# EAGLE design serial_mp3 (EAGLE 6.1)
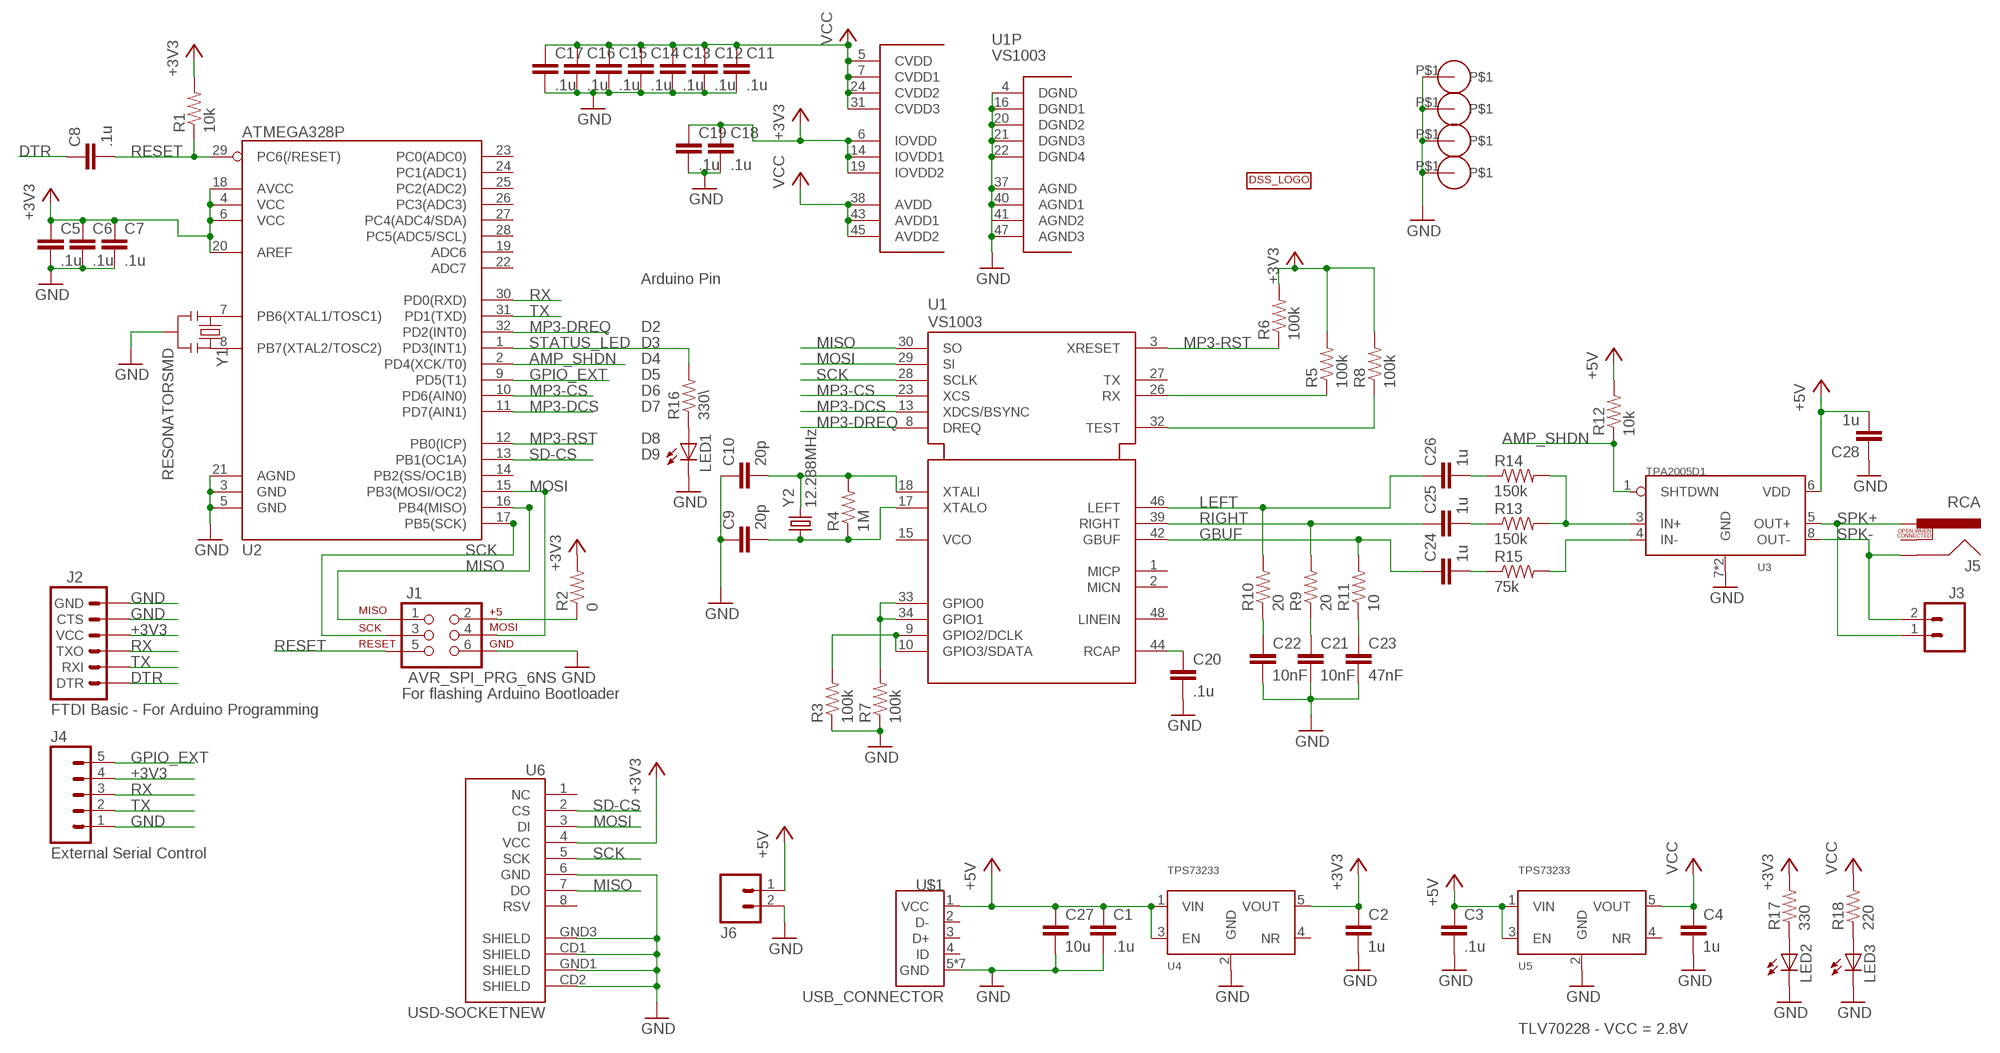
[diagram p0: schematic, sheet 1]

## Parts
C1  .1u  CAP0603-CAP  [0603-CAP]
C2  1u  CAP0603-CAP  [0603-CAP]
C3  .1u  CAP0603-CAP  [0603-CAP]
C4  1u  CAP0603-CAP  [0603-CAP]
C5  .1u  CAP0603-CAP  [0603-CAP]
C6  .1u  CAP0603-CAP  [0603-CAP]
C7  .1u  CAP0603-CAP  [0603-CAP]
C8  .1u  CAP0603-CAP  [0603-CAP]
C9  20p  CAP0603-CAP  [0603-CAP]
C10  20p  CAP0603-CAP  [0603-CAP]
C11  .1u  CAP0603-CAP  [0603-CAP]
C12  .1u  CAP0603-CAP  [0603-CAP]
C13  .1u  CAP0603-CAP  [0603-CAP]
C14  .1u  CAP0603-CAP  [0603-CAP]
C15  .1u  CAP0603-CAP  [0603-CAP]
C16  .1u  CAP0603-CAP  [0603-CAP]
C17  .1u  CAP0603-CAP  [0603-CAP]
C18  .1u  CAP0603-CAP  [0603-CAP]
C19  .1u  CAP0603-CAP  [0603-CAP]
C20  .1u  CAP0603-CAP  [0603-CAP]
C21  10nF  CAP0603-CAP  [0603-CAP]
C22  10nF  CAP0603-CAP  [0603-CAP]
C23  47nF  CAP0603-CAP  [0603-CAP]
C24  1u  CAP0603-CAP  [0603-CAP]
C25  1u  CAP0603-CAP  [0603-CAP]
C26  1u  CAP0603-CAP  [0603-CAP]
C27  10u  CAP0603-CAP  [0603-CAP]
C28  1u  CAP0603-CAP  [0603-CAP]
J1  AVR_SPI_PRG_6NS  [2X3-NS]
J2  ARDUINO_SERIAL_PROGRAMPTH  [1X06]
J3  M02PTH  [1X02]
J4  M05PTH  [1X05]
J5  RCA  [RCA]
J6  M02PTH  [1X02]
LED1  LED0603  [LED-0603]
LED2  LED0603  [LED-0603]
LED3  LED0603  [LED-0603]
R1  10k  RESISTOR0603-RES  [0603-RES]
R2  0  RESISTOR0603-RES  [0603-RES]
R3  100k  RESISTOR0603-RES  [0603-RES]
R4  1M  RESISTOR0603-RES  [0603-RES]
R5  100k  RESISTOR0603-RES  [0603-RES]
R6  100k  RESISTOR0603-RES  [0603-RES]
R7  100k  RESISTOR0603-RES  [0603-RES]
R8  100k  RESISTOR0603-RES  [0603-RES]
R9  20  RESISTOR0603-RES  [0603-RES]
R10  20  RESISTOR0603-RES  [0603-RES]
R11  10  RESISTOR0603-RES  [0603-RES]
R12  10k  RESISTOR0603-RES  [0603-RES]
R13  150k  RESISTOR0603-RES  [0603-RES]
R14  150k  RESISTOR0603-RES  [0603-RES]
R15  75k  RESISTOR0603-RES  [0603-RES]
R16  330\  RESISTOR0603-RES  [0603-RES]
R17  330  RESISTOR0603-RES  [0603-RES]
R18  220  RESISTOR0603-RES  [0603-RES]
U1  VS1003  [LQFP48]
U2  ATMEGA328P  ATMEGA328_SMT  [TQFP32-08]
U3  TPA2005D1  [S-PDSO-G08]
U4  TPS73233  [SOT23-5]
U5  TPS73233  [SOT23-5]
U6  USD-SOCKETNEW  [MICRO-SD-SOCKET-PP]
U$1  USB_CONNECTOR  [USB_MICRO]
U$2  DSSTOP  [DSS]
U$3  GNDHOLE  [GNDHOLE]
U$4  GNDHOLE  [GNDHOLE]
U$5  GNDHOLE  [GNDHOLE]
U$6  GNDHOLE  [GNDHOLE]
Y1  RESONATORSMD  [RESONATOR-SMD]
Y2  12.288MHz  NX3225GA  [SMD-4_3]

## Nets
+3V3: C2.1 C5.1 C6.1 C7.1 C18.1 C19.1 J2.4(VCC) J4.4 R1.2 R2.2 R5.2 R6.2 R8.2 R17.2 U1.6(IOVDD) U1.14(IOVDD1) U1.19(IOVDD2) U2.4(VCC) U2.6(VCC) U2.18(AVCC) U2.20(AREF) U4.5(VOUT) U6.4(VCC)
+5V: C1.1 C3.1 C27.1 C28.2 J6.1 R12.2 U3.6(VDD) U4.1(VIN) U4.3(EN) U5.1(VIN) U5.3(EN) U$1.1(VCC)
AMP_SHDN: R12.1 U2.2(PD4(XCK/T0)) U3.1(SHTDWN)
DTR: C8.1 J2.1(DTR)
GBUF: C24.1 R11.2 U1.42(GBUF)
GND: C1.2 C2.2 C3.2 C4.2 C5.2 C6.2 C7.2 C9.1 C10.1 C11.2 C12.2 C13.2 C14.2 C15.2 C16.2 C17.2 C18.2 C19.2 C20.2 C21.2 C22.2 C23.2 C27.2 C28.1 J1.6 J2.5(CTS) J2.6(GND) J4.1 J6.2 LED1.C LED2.C LED3.C R3.1 R7.1 U1.4(DGND) U1.16(DGND1) U1.20(DGND2) U1.21(DGND3) U1.22(DGND4) U1.37(AGND) U1.40(AGND1) U1.41(AGND2) U1.47(AGND3) U2.3(GND) U2.5(GND) U2.21(AGND) U3.7(GND) U3.TH(GND) U4.2(GND) U5.2(GND) U6.6(GND) U6.CD1(SHIELD) U6.CD2(SHIELD) U6.GND1(SHIELD) U6.GND3(SHIELD) U$1.5(GND) U$1.GND1(GND) U$1.GND2(GND) U$1.GND3(GND) U$1.GND4(GND) U$1.GND5(GND) U$1.GND6(GND) U$3.P$1 U$4.P$1 U$5.P$1 U$6.P$1 Y1.2
GPIO_EXT: J4.5 U2.9(PD5(T1))
LEFT: C26.1 R10.2 U1.46(LEFT)
MISO: J1.1 U1.30(SO) U2.16(PB4(MISO)) U6.7(DO)
MOSI: J1.4 U1.29(SI) U2.15(PB3(MOSI/OC2)) U6.3(DI)
MP3-CS: U1.23(XCS) U2.10(PD6(AIN0))
MP3-DCS: U1.13(XDCS/BSYNC) U2.11(PD7(AIN1))
MP3-DREQ: U1.8(DREQ) U2.32(PD2(INT0))
MP3-RST: R6.1 U1.3(XRESET) U2.12(PB0(ICP))
N$1: J1.2 R2.1
N$2: C10.2 R4.2 U1.18(XTALI) Y2.3
N$3: C9.2 R4.1 U1.17(XTALO) Y2.1
N$4: R7.2 U1.33(GPIO0) U1.34(GPIO1)
N$5: U2.8(PB7(XTAL2/TOSC2)) Y1.3
N$6: U2.7(PB6(XTAL1/TOSC1)) Y1.1
N$7: R5.1 U1.26(RX)
N$8: R8.1 U1.32(TEST)
N$9: C20.1 U1.44(RCAP)
N$10: C23.1 R11.1
N$11: C22.1 R10.1
N$12: C21.1 R9.1
N$13: C24.2 R15.1
N$14: C25.2 R13.1
N$15: C26.2 R14.1
N$16: R13.2 R14.2 U3.3(IN+)
N$17: R15.2 U3.4(IN-)
N$18: R3.2 U1.9(GPIO2/DCLK) U1.10(GPIO3/SDATA)
N$20: LED2.A R17.1
N$21: LED1.A R16.1
N$22: LED3.A R18.1
RESET: C8.2 J1.5 R1.1 U2.29(PC6(/RESET))
RIGHT: C25.1 R9.2 U1.39(RIGHT)
RX: J2.3(TXO) J4.3 U2.30(PD0(RXD))
SCK: J1.3 U1.28(SCLK) U2.17(PB5(SCK)) U6.5(SCK)
SD-CS: U2.13(PB1(OC1A)) U6.2(CS)
SPK+: J3.1 J5.PIN U3.5(OUT+)
SPK-: J3.2 J5.SHELL U3.8(OUT-)
STATUS_LED: R16.2 U2.1(PD3(INT1))
TX: J2.2(RXI) J4.2 U2.31(PD1(TXD))
VCC: C4.1 C11.1 C12.1 C13.1 C14.1 C15.1 C16.1 C17.1 R18.2 U1.5(CVDD) U1.7(CVDD1) U1.24(CVDD2) U1.31(CVDD3) U1.38(AVDD) U1.43(AVDD1) U1.45(AVDD2) U5.5(VOUT)
Unconnected: J5.SWITCH U1.1(MICP) U1.2(MICN) U1.15(VCO) U1.27(TX) U1.48(LINEIN) U2.14(PB2(SS/OC1B)) U2.19(ADC6) U2.22(ADC7) U2.23(PC0(ADC0)) U2.24(PC1(ADC1)) U2.25(PC2(ADC2)) U2.26(PC3(ADC3)) U2.27(PC4(ADC4/SDA)) U2.28(PC5(ADC5/SCL)) U4.4(NR) U5.4(NR) U6.1(NC) U6.8(RSV) U$1.2(D-) U$1.3(D+) U$1.4(ID)

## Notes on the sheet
- Arduino Pin
- D2
- D3
- D4
- D5
- D6
- D7
- D8
- D9
- For flashing Arduino Bootloader
- FTDI Basic - For Arduino Programming
- External Serial Control
- TLV70228 - VCC = 2.8V

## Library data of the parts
C1-C28 = SparkFun-Passives:CAP: Capacitor
J1 = SparkFun-Connectors:AVR_SPI_PRG_6: AVR ISP 6 Pin This is the reduced ISP connector for AVR programming. Common on Arduino. This footprint will take up less PCB space and can be used with a 10-pin to 6-pin adapter such as SKU: BOB-08508
J2 = SparkFun-Connectors:ARDUINO_SERIAL_PROGRAM: FTDI connector footprints
J3 J6 = SparkFun-Connectors:M02: Header 2
J4 = SparkFun-Connectors:M05: Header 5 Standard 5-pin 0.1" header. Use with straight break away headers (SKU : PRT-00116), right angle break away headers (PRT-00553), swiss pins (PRT-00743), machine pins (PRT-00117), and female headers (PRT-00115). Molex polarized connector foot print use with SKU : PRT-08230 with associated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
J5 = SparkFun-Connectors:RCA
LED1-LED3 = SparkFun-LED:LED: LEDs
R1-R18 = SparkFun-Passives:RESISTOR: Resistor
U1 = vlsi-web:VS1003: MP3 / WMA / MIDI Audio Codec Circuit
U2 = SparkFun-DigitalIC:ATMEGA328_SMT: 32-Pin Atmega328 part Commonly used on Arduino compatible boards Available in QFP and QFN packages TQFP is IC-09069 QFN is non-stock; PROD_ID: IC-09069
U3 = DSS:TPA2005D1: TI TPA2005D1 1.4 W mono class D audio amp
U4 U5 = DSS:TPS73233: TI TPS73233 - fixed output http://www.ti.com/product/tps73233
U6 = SparkFun-Connectors:USD-SOCKET: microSD Socket Push-push type uSD socket. Schematic element and footprint production proven. Spark Fun Electronics SKU : PRT-00127. tDoc lines correctly indicate media card edge positions when inserting (unlocked, locked, depressed).
U$1 = DSS:USB_CONNECTOR: USB Connector http://www.digikey.com/product-detail/en/10118192-0001LF/609-4613-1-ND/2785378
U$2 = DSS:DSS: DSS LOGO
U$3-U$6 = GT-IEEE:GNDHOLE
Y1 = SparkFun-FreqCtrl:RESONATOR: Resonator Small SMD resonator. This is the itty bitty 10/20MHz resonators with built in caps. CSTCE10M0G55 and CSTCE20M0V53. Footprint has been reviewed closely but hasn't been tested yet.
Y2 = DSS:NX3225GA: NX3225GA 26 MHz SMD crystal

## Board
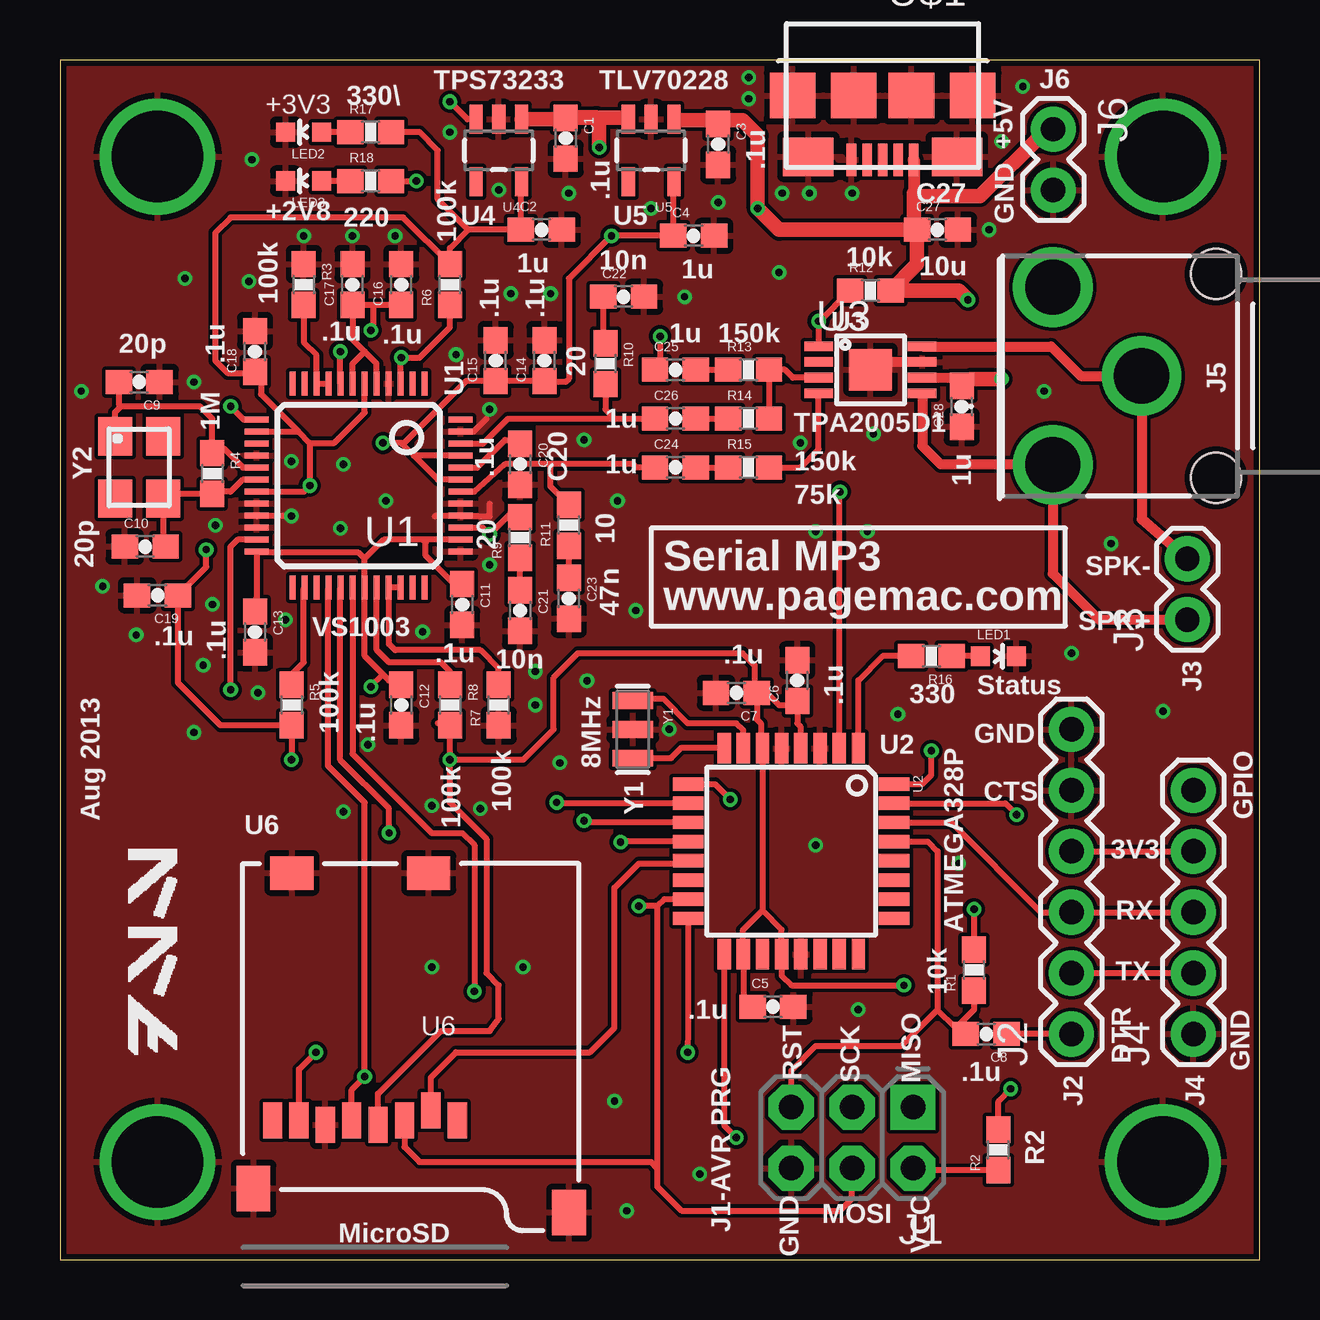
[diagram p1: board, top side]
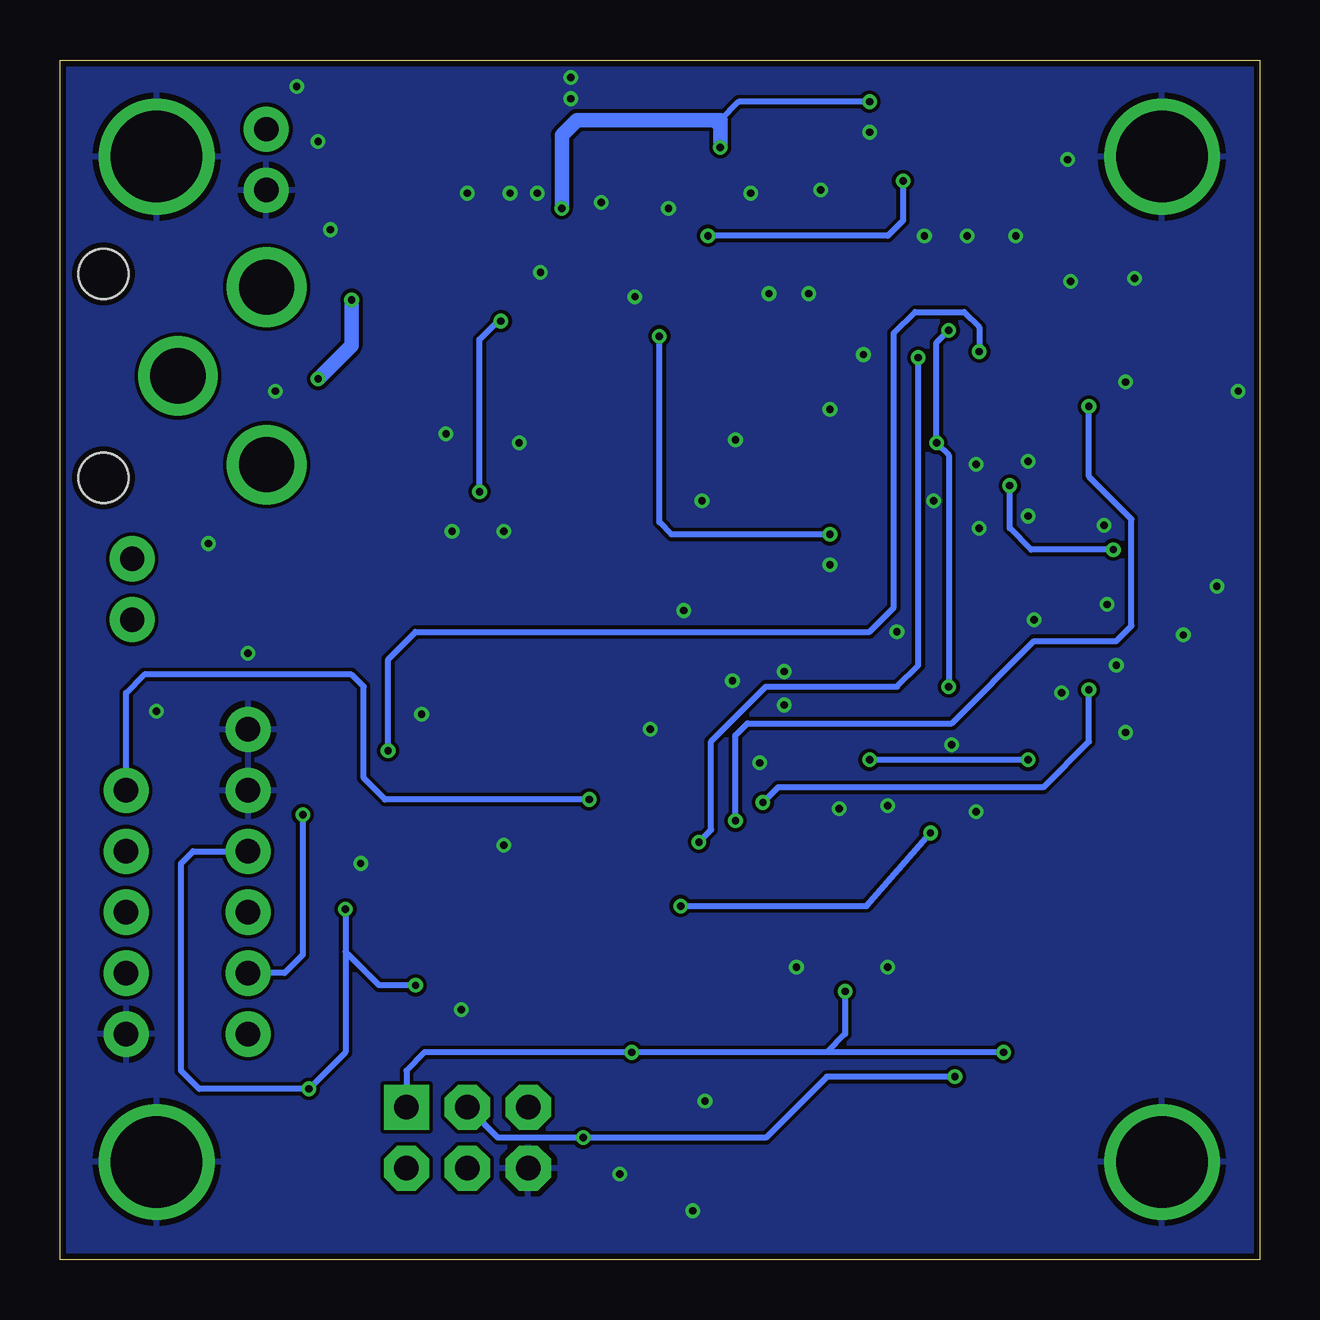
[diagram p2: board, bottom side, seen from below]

Size 50 x 50 mm. Coordinates in mm from the lower left corner, seen from the top.
Outline: 0,0 50,0 50,50 0,50 0,0
Copper layers (1*16): Top 0.035mm / dielectric 1.5mm / Bottom 0.035mm
Design rules: minimum track width 6mil, minimum drill 12mil, track to track 6mil, track to pad 6mil, pad to pad 6mil, via to via 6mil, smd to smd 0mil, copper to edge 10mil, drill to drill 10mil, minimum pad ring 10mil, minimum via ring 6mil, stop-mask expansion 2mil, vias tented up to drill 100mil, thermal gap 10mil

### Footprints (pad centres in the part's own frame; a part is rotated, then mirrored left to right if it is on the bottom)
0603-CAP = smd 1.1 x 1: 1 -0.85,0; 2 0.85,0
2X3-NS = drill 1.016 pad 1.88 square: 1 -2.54,-1.27 | drill 1.016 pad 1.88 octagon: 2 -2.54,1.27; 3 0,-1.27; 4 0,1.27; 5 2.54,-1.27; 6 2.54,1.27
1X06 = drill 1.016 pad 1.88: 1 0,0; 2 2.54,0; 3 5.08,0; 4 7.62,0; 5 10.16,0; 6 12.7,0
1X02 = drill 1.016 pad 1.88: 1 0,0; 2 2.54,0
1X05 = drill 1.016 pad 1.88: 1 0,0; 2 2.54,0; 3 5.08,0; 4 7.62,0; 5 10.16,0
RCA = drill 2.3: PIN 3.7,3.7; SHELL 0,0; SWITCH 3.7,-3.7 | hole 2.1: -3.1,4.25; -3.1,-4.25
LED-0603 = smd 0.8 x 0.8: A 0,-0.75; C 0,0.75
0603-RES = smd 1.1 x 1: 1 -0.85,0; 2 0.85,0
LQFP48 = smd 0.25 x 1: 1 -2.75,-4.25; 2 -2.25,-4.25; 3 -1.75,-4.25; 4 -1.25,-4.25; 5 -0.75,-4.25; 6 -0.25,-4.25; 7 0.25,-4.25; 8 0.75,-4.25; 9 1.25,-4.25; 10 1.75,-4.25; 11 2.25,-4.25; 12 2.75,-4.25; 25 2.75,4.25; 26 2.25,4.25; 27 1.75,4.25; 28 1.25,4.25; 29 0.75,4.25; 30 0.25,4.25; 31 -0.25,4.25; 32 -0.75,4.25; 33 -1.25,4.25; 34 -1.75,4.25; 35 -2.25,4.25; 36 -2.75,4.25 | smd 1 x 0.25: 13 4.25,-2.75; 14 4.25,-2.25; 15 4.25,-1.75; 16 4.25,-1.25; 17 4.25,-0.75; 18 4.25,-0.25; 19 4.25,0.25; 20 4.25,0.75; 21 4.25,1.25; 22 4.25,1.75; 23 4.25,2.25; 24 4.25,2.75; 37 -4.25,2.75; 38 -4.25,2.25; 39 -4.25,1.75; 40 -4.25,1.25; 41 -4.25,0.75; 42 -4.25,0.25; 43 -4.25,-0.25; 44 -4.25,-0.75; 45 -4.25,-1.25; 46 -4.25,-1.75; 47 -4.25,-2.25; 48 -4.25,-2.75
TQFP32-08 = smd 1.27 x 0.559: 1 -4.293,2.8; 2 -4.293,2; 3 -4.293,1.2; 4 -4.293,0.4; 5 -4.293,-0.4; 6 -4.293,-1.2; 7 -4.293,-2; 8 -4.293,-2.8; 17 4.293,-2.8; 18 4.293,-2; 19 4.293,-1.2; 20 4.293,-0.4; 21 4.293,0.4; 22 4.293,1.2; 23 4.293,2; 24 4.293,2.8 | smd 0.559 x 1.27: 9 -2.8,-4.293; 10 -2,-4.293; 11 -1.2,-4.293; 12 -0.4,-4.293; 13 0.4,-4.293; 14 1.2,-4.293; 15 2,-4.293; 16 2.8,-4.293; 25 2.8,4.293; 26 2,4.293; 27 1.2,4.293; 28 0.4,4.293; 29 -0.4,4.293; 30 -1.2,4.293; 31 -2,4.293; 32 -2.8,4.293
S-PDSO-G08 = smd 0.4 x 1.2: 1 -0.975,-2.157; 2 -0.325,-2.157; 3 0.325,-2.157; 4 0.975,-2.157; 5 0.975,2.157; 6 0.325,2.157; 7 -0.325,2.157; 8 -0.975,2.157 | smd 1.73 x 1.78: TH 0,0
SOT23-5 = smd 0.55 x 1.2: 1 -0.95,-1.3; 2 0,-1.3; 3 0.95,-1.3; 4 0.95,1.3; 5 -0.95,1.3
MICRO-SD-SOCKET-PP = smd 0.8 x 1.5: 1 -8.94,10.7; 2 -7.84,10.3; 3 -6.74,10.7; 4 -5.64,10.9; 5 -4.54,10.7; 6 -3.44,10.9; 7 -2.34,10.7; 8 -1.24,10.7 | smd 1.8 x 1.4: CD1 -2.05,0.4; CD2 -7.75,0.4 | smd 1.4 x 1.9: GND1 -13.6,14.55; GND3 -0.45,13.55
USB_MICRO = smd 0.4 x 1.35: 1 -1.3,2.675; 2 -0.65,2.675; 3 0,2.675; 4 0.65,2.675; 5 1.3,2.675 | smd 1.9 x 1.9: GND1 -3.75,0; GND2 -1.2,0; GND3 1.2,0; GND4 3.75,0 | smd 2.1 x 1.6: GND5 -3.1,2.55; GND6 3.1,2.55
GNDHOLE = drill 3.81: P$1 0,0
RESONATOR-SMD = smd 0.7 x 1.7: 1 -1.2,0; 2 0,0; 3 1.2,0
SMD-4_3 = smd 1.6 x 1.4: 1 -1.3,-1; 2 1.3,-1; 3 1.3,1; 4 -1.3,1

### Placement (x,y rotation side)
C1  21.08,46.74 270 top
C2  20.07,42.93 0 top
C3  27.43,46.48 270 top
C4  26.42,42.67 0 top
C5  29.72,10.54 0 top
C6  30.73,24.13 90 top
C7  28.19,23.62 180 top
C8  38.61,9.4 180 top
C9  3.3,36.58 180 top
C10  3.56,29.72 0 top
C11  16.76,27.3 270 top
C12  14.22,23.11 270 top
C13  8.13,26.16 270 top
C14  20.19,37.47 90 top
C15  18.16,37.47 90 top
C16  14.22,40.64 90 top
C17  12.19,40.64 90 top
C18  8.13,37.85 90 top
C19  4.06,27.69 180 top
C20  19.18,33.15 270 top
C21  19.18,27.05 270 top
C22  23.5,40.13 0 top
C23  21.21,27.56 270 top
C24  25.65,33.02 0 top
C25  25.65,37.08 0 top
C26  25.65,35.05 0 top
C27  36.58,42.93 0 top
C28  37.59,35.56 90 top
J1  33.02,5.08 180 top
J2  42.16,9.4 90 top
J3  46.99,26.67 90 top
J4  47.24,9.4 90 top
J5  45.09,36.83 180 top
J6  41.4,47.12 270 top
LED1  39.12,25.15 270 top
LED2  10.16,46.99 90 top
LED3  10.16,44.96 90 top
R1  38.1,12.06 90 top
R2  39.12,4.57 90 top
R3  10.16,40.64 270 top
R4  6.35,32.77 270 top
R5  9.65,23.11 270 top
R6  16.26,40.64 90 top
R7  18.29,23.11 90 top
R8  16.26,23.11 270 top
R9  19.18,30.1 90 top
R10  22.73,37.34 270 top
R11  21.21,30.61 90 top
R12  33.78,40.39 0 top
R13  28.7,37.08 0 top
R14  28.7,35.05 0 top
R15  28.7,33.02 0 top
R16  36.32,25.15 180 top
R17  12.95,46.99 0 top
R18  12.95,44.96 0 top
U1  12.45,32.26 180 top
U2  30.48,17.02 270 top
U3  33.78,37.08 270 top
U4  18.29,46.23 180 top
U5  24.64,46.23 180 top
U6  7.62,16.51 180 top
U$1  34.29,48.51 180 top
U$2  5.08,8.38 90 top
U$3  45.97,4.06 0 top
U$4  4.06,4.06 0 top
U$5  4.06,45.97 0 top
U$6  45.97,45.97 0 top
Y1  23.88,22.1 270 top
Y2  3.3,33.02 270 top

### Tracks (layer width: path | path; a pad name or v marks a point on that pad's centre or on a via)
+3V3  (via drill 0.3)
  Top 0.254: 29.28,14.55 U2.6 29.21,21.38 29.21,22.35 29.04,22.52 C7.1 29.08,23.62 | 29.28,14.55 28.45,13.72 28.45,12.76 U2.18 28.48,10.68 C5.1 | 29.28,14.55 30.08,13.75 U2.20 30.08,11.83 30.48,11.43 v35.18,11.43 | J2.4 J4.4 | R2.2 39.12,6.6 v39.62,7.11 | v38.1,14.61 R1.2 38.1,12.83 | U1.14 9.94,34.51 | 9.94,34.51 10.41,34.04 | 10.41,34.04 v10.41,32.26 10.16,32 U1.19 | 10.41,34.04 11.43,34.04 12.7,35.31 U1.6 | U6.4 13.26,6.91 15.88,9.53 17.91,9.53 18.29,10.03 18.29,11.43 17.78,11.94 17.78,17.53 16.26,19.05 v16.26,20.83 | U4.5 19.22,44.91 C2.1 17.02,42.93 | 17.02,42.93 15.75,44.2 15.75,46.23 14.99,46.99 R17.2 | v9.65,20.83 R5.2 6.69,22.26 4.91,24.04 C19.1 6.1,28.87 v6.1,29.59 | 15.75,22.35 R8.2 v16.26,20.83 | 17.02,42.93 16.26,42.16 R6.2 14.31,43.43 7.11,43.43 6.48,42.8 6.48,37.47 6.99,36.96 8.38,36.96 | U2.4 30.86,21.33 30.86,22.23 30.73,22.35 C6.1 30.57,23.11 29.97,23.11 29.46,23.62 29.08,23.62 | C18.1 8.38,36.96 | 8.38,36.96 8.38,36.07 9.94,34.51 | v16.26,20.83 19.3,20.83 20.57,22.1 20.57,24.26 21.59,25.27 28.45,25.27 28.96,24.77 28.96,23.75 29.08,23.62
  Bottom 0.254: J2.4 44.45,17.02 44.96,16.51 44.96,7.87 44.2,7.11 v39.62,7.11 38.1,8.64 38.1,12.83 | v38.1,14.61 38.1,12.83 | v6.1,29.59 9.53,29.59 10.41,30.48 v10.41,32.26 | v9.65,20.83 v16.26,20.83 | v35.18,11.43 36.7,11.43 38.1,12.83
+5V  (via drill 0.3)
  Top 0.254: 35.59,43.32 C27.1 | 27.6,47.5 C3.1 | 21.08,47.5 21.05,47.53 21.05,47.56 C1.1 | 23.63,47.59 U5.3 | J6.1 41.02,46.99 | 35.72,44.32 35.59,44.45 | U4.3 16.99,47.53 v16.26,48.26 | 25.65,47.5 25.62,47.5 U5.1
  Top 0.406: U3.6 38.01,36.76 C28.2
  Top 0.508: U$1.1 35.59,44.45
  Top 0.61: 35.59,44.45 35.59,43.32 | 27.6,47.5 28.45,47.5 29.08,46.86 v29.08,43.81 29.97,42.93 C27.1 35.73,41.48 R12.2 37.47,40.39 v37.85,40.01 | U4.1 21.05,47.53 | 23.63,47.59 C1.1 21.12,47.62 22.35,47.62 22.48,47.5 v22.48,46.35 | 41.02,46.99 38.35,44.32 35.72,44.32 | C3.1 27.27,47.5 25.65,47.5 | v39.24,36.7 37.97,36.7 C28.2
  Bottom 0.254: v16.26,48.26 21.72,48.26 22.48,47.5 22.73,47.24
  Bottom 0.61: v22.48,46.35 22.48,47.5 28.45,47.5 29.08,46.86 v29.08,43.81 | v37.85,40.01 37.85,38.1 v39.24,36.7
AMP_SHDN  (via drill 0.3)
  Top 0.254: U3.1 31.62,39.08 | 31.62,39.08 R12.1 | U2.2 32.48,31.97 v32.51,32 | 31.62,39.08 v31.62,39.11 v31.62,39.12
  Bottom 0.254: v32.51,32 32.51,38.35 31.71,39.16 31.67,39.16 v31.62,39.12
DTR
  Top 0.254: J2.1 C8.1
GBUF
  Top 0.254: U1.42 17.28,32.01 18.54,33.15 20.45,33.15 | C24.1 24,33.02 23.88,33.15 20.45,33.15 | R11.2 20.45,32.22 20.45,33.15
GND  (via drill 0.3)
  Top 0.254: U1.47 17.24,34.51 17.78,35.05 | v9.65,30.99 8.22,30.99 U1.21 | U1.40 16.72,30.99 | 16.72,30.99 17.91,30.99 17.91,31.5 | 16.72,30.99 15.62,30.99
  Top 0.406: U3.7 33.98,37.41 U3.TH
  other vias: 19.3,12.19 7.87,40.77 33.66,30.35 23.11,6.6 33.27,10.41 37.47,16.51 8,45.85 5.21,40.89 38.73,42.93 29.97,41.15 20.83,20.7 31.5,17.27 45.97,22.86 3.17,26.04 23.62,2.03 15.49,18.92 25.4,22.1 15.49,12.19 9.65,33.27 13.59,31.62 15.11,26.16 21.97,24.13 30.86,34.04 21.84,34.16 23.24,31.62 17.91,35.43 20.45,40.26 18.8,40.26 13.97,42.67 12.19,42.67 10.16,42.67 31.24,44.45 28.7,49.28 39.24,46.61 6.48,30.61 6.35,27.3 1.78,28.07 5.59,36.58 0.89,36.2 8.26,23.62 21.21,44.45 18.29,44.58 16.26,46.99 24.64,43.81 27.43,44.07 26.04,40.13 12.83,21.46 17.53,18.8 26.67,3.56 19.81,24.51 24,27.05 17.91,28.96 11.81,33.15 16.51,37.72 5.59,21.97 11.81,18.67 11.68,30.48 5.97,24.77 41.02,36.2 31.5,30.35 43.81,29.84 42.16,25.27 34.92,22.73 33.02,44.45 40.13,48.9 28.7,48.39 30.1,44.45 33.91,34.42 19.81,23.11 9.4,26.67
  pour Bottom: 0,50.04 50.04,50.04 50.04,0 0,0
  pour Top: 0,50.04 50.04,50.04 50.04,0 0,0
GPIO_EXT  (via drill 0.3)
  Top 0.254: U2.9 27.3,19.82 v27.94,19.18
  Bottom 0.254: v27.94,19.18 36.45,19.18 37.34,20.07 37.34,23.88 37.85,24.38 46.48,24.38 47.24,23.62 J4.5
LEFT
  Top 0.254: U1.46 17.62,34.01 18.67,35.05 23.11,35.05 | 23.11,35.05 C26.1 | R10.2 22.73,35.43 23.11,35.05
MISO  (via drill 0.3)
  Top 0.254: U2.16 26.19,9.63 v26.16,8.64 | U6.7 9.96,7.93 v10.67,8.64 | U1.30 12.2,26.16 12.19,21.08 15.49,17.78 16.76,17.78 17.27,17.27 v17.27,11.18
  Bottom 0.254: J1.1 35.56,7.87 34.8,8.64 v26.16,8.64 18.03,8.64 | v10.67,8.64 18.03,8.64 | v17.27,11.18 17.27,9.4 18.03,8.64
MOSI  (via drill 0.3)
  Top 0.254: U2.15 25.18,15.02 24.89,14.73 | 24.89,14.73 24.89,3.81 | 24.89,3.81 24.89,3.05 25.91,2.03 32.51,2.03 33.02,2.54 J1.4 | U6.3 14.36,4.69 14.99,4.06 24.64,4.06 24.89,3.81 | 24.89,14.73 v24.13,14.73 | v13.72,17.78 13.72,18.8 11.68,20.83 11.68,28 U1.29
  Bottom 0.254: v24.13,14.73 16.38,14.73 v13.72,17.78
MP3-CS  (via drill 0.3)
  Top 0.254: U2.10 20.73,19.02 v20.7,19.05 | v7.11,23.75 7.11,29.72 7.4,30.01 U1.23
  Bottom 0.254: v7.11,23.75 7.11,21.59 9.02,19.68 20.07,19.68 v20.7,19.05
MP3-DCS  (via drill 0.3)
  Top 0.254: U2.11 21.9,18.22 v21.84,18.29 | U1.13 7.66,35.01 v7.11,35.56
  Bottom 0.254: v21.84,18.29 21.84,21.84 21.34,22.35 12.83,22.35 9.4,25.78 5.97,25.78 5.33,26.42 5.33,30.86 7.11,32.64 v7.11,35.56
MP3-DREQ  (via drill 0.3)
  Top 0.254: U2.32 35.95,19.82 36.32,20.19 v36.32,21.21 | U1.8 11.68,36.52 v11.68,37.85
  Bottom 0.254: v36.32,21.21 36.32,25.02 35.18,26.16 16.26,26.16 15.24,27.18 15.24,38.61 14.35,39.5 12.32,39.5 11.68,38.86 v11.68,37.85
MP3-RST  (via drill 0.3)
  Top 0.254: U2.12 23.39,17.42 v23.37,17.4 | U1.3 14.2,37.56 v14.22,37.59 14.99,37.59 16.26,38.86 R6.1
  Bottom 0.254: v23.37,17.4 22.86,17.91 22.86,21.59 20.57,23.88 15.11,23.88 14.22,24.77 v14.22,37.59
N$1
  Top 0.254: R2.1 35.65,3.72 J1.2
N$2
  Top 0.254: U1.18 7.62,32.51 7.11,32 6.44,32 R4.2 4.5,31.92 Y2.3 4.3,29.57 C10.2
N$3
  Top 0.254: U1.17 7.63,33.01 6.86,33.78 6.52,33.78 R4.1 6.35,35.05 5.84,35.56 2.54,35.56 | 2.54,35.56 2.29,35.31 2.29,34.34 Y2.1 | C9.2 2.45,35.65 2.54,35.56
N$4
  Top 0.254: U1.34 U1.33 13.7,27.96 13.72,27.94 13.72,25.65 13.97,25.4 17.53,25.4 18.29,24.64 R7.2
N$5
  Top 0.254: U2.8 27.66,21.34 25.91,21.34 25.47,20.9 Y1.3
N$6
  Top 0.254: U2.7 28.48,22.07 28.19,22.35 26.16,22.35 25.15,23.37 23.95,23.37 Y1.1
N$7
  Top 0.254: R5.1 9.65,24.38 10.16,24.89 10.16,27.97 U1.26
N$8
  Top 0.254: R8.1 16.26,24.51 15.88,24.89 13.72,24.89 13.21,25.4 13.21,28 U1.32
N$9
  Top 0.254: U1.44 17.39,33.01 18.54,34.16 19.27,34.16 C20.1
N$10
  Top 0.254: C23.1 R11.1
N$11
  Top 0.254: C22.1 22.64,38.28 R10.1
N$12
  Top 0.254: C21.1 R9.1
N$13
  Top 0.254: C24.2 R15.1
N$14
  Top 0.254: C25.2 R13.1
N$15
  Top 0.254: C26.2 R14.1
N$16
  Top 0.254: R14.2 R13.2 30.23,37.08 30.55,36.76 U3.3
N$17
  Top 0.254: R15.2 30.86,33.02 31.62,33.78 U3.4
N$18
  Top 0.254: R3.2 10.16,38.23 10.7,37.69 U1.10 U1.9
N$20
  Top 0.254: R17.1 LED2.A
N$21
  Top 0.254: LED1.A R16.1
N$22
  Top 0.254: R18.1 LED3.A
RESET
  Top 0.254: U2.29 36.18,17.42 36.58,17.02 36.58,10.41 | 36.58,10.41 35.05,8.89 31.5,8.89 30.48,7.87 J1.5 | C8.2 37.59,9.4 37.34,9.65 | 37.34,9.65 36.58,10.41 | R1.1 38.1,10.41 37.34,9.65
RIGHT  (via drill 0.3)
  Top 0.254: U1.39 17.62,30.51 v17.91,30.23 18.76,31.08 R9.2 | v25.02,38.48 25.02,37.34 24.8,37.12 | 24.8,37.12 24.77,37.08 | C25.1 24.8,37.12
  Bottom 0.254: v17.91,30.23 24.51,30.23 25.02,30.73 v25.02,38.48
RX
  Top 0.254: U2.30 37.15,18.22 40.89,14.48 J2.3 J4.3
SCK  (via drill 0.3)
  Top 0.254: U2.17 27.68,5.59 v28.19,5.08 | U6.5 12.16,7.08 v12.7,7.62 12.7,19.05 11.18,20.57 11.18,27.94 11.2,27.96 U1.28
  Bottom 0.254: J1.3 31.75,5.08 v28.19,5.08 20.57,5.08 18.03,7.62 v12.7,7.62
SD-CS
  Top 0.254: U6.2 15.46,7.59 16.51,8.64 22.1,8.64 23.11,9.65 23.11,15.49 24.13,16.51 26.08,16.51 U2.13
SPK+
  Top 0.406: U3.5 35.94,33.91 36.7,33.15 41.49,33.15 J5.PIN 41.38,28.59 43.31,26.67 J3.1
SPK-
  Top 0.406: U3.8 41.32,38.06 42.55,36.83 J5.SHELL 45.09,30.86 J3.2
STATUS_LED
  Top 0.254: U2.1 33.28,24.14 34.29,25.15 R16.2
TX  (via drill 0.3)
  Top 0.254: J2.2 J4.2 | U2.31 39.4,19.02 v39.88,18.54
  Bottom 0.254: v39.88,18.54 39.88,12.7 40.64,11.94 J2.2
VCC  (via drill 0.3)
  Top 0.254: U5.5 25.57,44.91 C4.1 v22.99,42.67 21.21,40.89 21.21,36.7 21.08,36.58 20.23,36.58 C14.1 C15.1 16.93,36.62 14.29,33.97 | C12.1 13.72,24.13 13.46,24.38 | 13.46,24.38 12.7,25.15 U1.31 12.7,29.21 | C13.1 8.2,27.59 U1.24 8.24,29.46 12.45,29.46 12.7,29.21 | U1.38 15.11,30.01 | 15.11,30.01 13.49,30.01 12.7,29.21 | 14.29,33.97 14.75,33.51 | U1.45 14.75,33.51 | U1.43 15.75,32.51 14.75,33.51 | C11.1 16.8,28.19 16.38,28.19 15.24,29.34 15.24,29.88 15.11,30.01 | U1.7 12.2,37.34 12.7,37.85 | 12.7,37.85 12.19,38.35 C17.1 13.08,39.79 | U1.5 13.2,37.35 12.7,37.85 | C16.1 13.08,39.79 | R18.2 v14.86,44.96 | 14.29,33.97 14.22,34.04 v13.46,34.04 | v12.95,38.73 13.08,38.86 13.08,39.79 | v12.95,23.88 13.46,24.38
  Bottom 0.254: v14.86,44.96 14.86,43.31 15.49,42.67 v22.99,42.67 | v12.95,38.73 13.46,38.23 v13.46,34.04 12.95,33.53 v12.95,23.88

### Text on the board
_tsilk: TPS73233 | TLV70228 | +3V3 | J6 | 330\ | .1u | .1u | +5V | +2V8 | U4 | U5 | C27 | 220 | GND | 100k | 100k | 1u | 10n | 1u | 10k | 10u | 20p | .1u | .1u | .1u | .1u | U3 | 20 | 1u | 150k | .1u | U1 | 1M | J5 | C20 | 1u | TPA2005D1 | Y2 | .1u | 1u | 150k | 1u | 75k | 20 | 10 | 20p | 47n | Serial MP3 | SPK- | .1u | VS1003 | www.pagemac.com | SPK+ | .1u | .1u | 100k | .1u | 10n | 330 | Status | J3 | .1u | 8MHz | .1u | GND | 100k | U2 | ATMEGA328P | GPIO | Y1 | CTS | U6 | 100k | Aug 2013 | 3V3 | RX | TX | 10k | DTR | .1u | RST | SCK | MISO | GND | .1u | J2 | J4 | R2 | GND | VCC | MicroSD | MOSI | J1-AVR PRG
